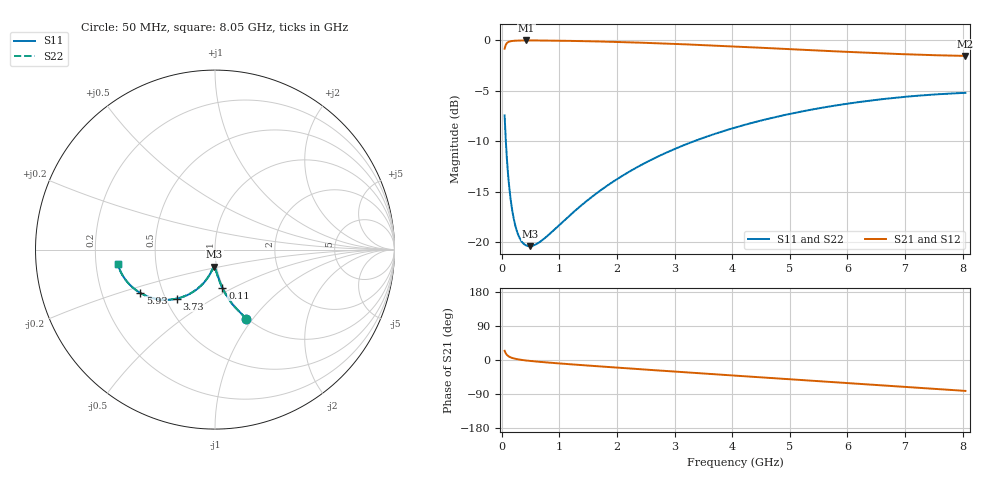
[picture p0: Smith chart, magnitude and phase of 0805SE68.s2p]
! AVX Thin Film Operation		Date: August 2001
! Description: Accu-P® Series, Thin Film, SMD, RF Capacitor
! Part Number: 08053K680FBT
! 50 MHz  -  8.05 GHz
! Serial Measurements
# mhz S db R 50
!	S11		S21		S12		S22
!	dB	Phase	dB	Phase	dB	Phase	dB	Phase
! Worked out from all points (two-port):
!   401 points, 50 MHz to 8.05 GHz, reference 50 ohm
!   highest |S21| = -0.04 dB at 430 MHz (marker M1); lowest = -1.6 dB at 8.05 GHz (marker M2)
!   |S21| within 3 dB of the highest: start of sweep to end of sweep
!   lowest |S11| = -20.4 dB at 490 MHz (marker M3), VSWR 1.21, Z = 48.8 - j9.4 ohm
!   |S11| at or under -10 dB: 71.27 MHz to 3.345 GHz (3.274 GHz wide, 192 % of centre)
!   |S22| runs from -20.4 to -5.2 dB; largest |S21 - S12| = 0
!   S11 on the Smith chart (normalised r, x): 50 MHz: 0.99, -0.93; 110 MHz: 0.99, -0.44; 3.73 GHz: 0.57, -0.35; 5.93 GHz: 0.37, -0.23; 8.05 GHz: 0.29, -0.07
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50  -7.46 -65.6  -0.86 24.3  -0.86 24.3  -7.46 -65.8
70  -9.88 -72.3  -0.47 17.6  -0.47 17.6  -9.88 -72.5
110  -13.30 -79.1  -0.21 10.7  -0.21 10.7  -13.30 -79.4
130  -14.53 -81.0  -0.16 8.7  -0.16 8.7  -14.53 -81.4
170  -16.40 -83.7  -0.10 6.0  -0.10 6.0  -16.40 -84.1
230  -18.23 -86.3  -0.07 3.3  -0.07 3.3  -18.23 -86.8
310  -19.58 -88.5  -0.05 1.0  -0.05 1.0  -19.58 -89.1
370  -20.10 -89.8  -0.04 -0.3  -0.04 -0.3  -20.10 -90.4
430  -20.34 -90.9  -0.04 -1.4  -0.04 -1.4  -20.34 -91.6
490  -20.40 -91.9  -0.04 -2.4  -0.04 -2.4  -20.40 -92.5
730  -19.68 -95.3  -0.05 -5.8  -0.05 -5.8  -19.68 -95.9
1390  -16.32 -103.2  -0.11 -13.5  -0.11 -13.5  -16.32 -103.6
2010  -13.73 -109.9  -0.19 -20.2  -0.19 -20.2  -13.73 -110.2
2730  -11.48 -117.5  -0.33 -27.7  -0.33 -27.7  -11.48 -117.7
3730  -9.23 -127.8  -0.56 -38.0  -0.56 -38.0  -9.23 -127.9
4050  -8.66 -131.0  -0.64 -41.2  -0.64 -41.2  -8.66 -131.2
4710  -7.68 -137.7  -0.82 -47.8  -0.82 -47.8  -7.68 -137.8
5390  -6.87 -144.5  -1.01 -54.6  -1.01 -54.6  -6.87 -144.5
5930  -6.36 -149.8  -1.16 -60.0  -1.16 -60.0  -6.36 -149.9
6730  -5.78 -157.8  -1.35 -68.0  -1.35 -68.0  -5.77 -157.9
7430  -5.42 -164.9  -1.49 -75.1  -1.49 -75.1  -5.42 -164.9
8050  -5.23 -171.4  -1.57 -81.5  -1.57 -81.5  -5.23 -171.4
